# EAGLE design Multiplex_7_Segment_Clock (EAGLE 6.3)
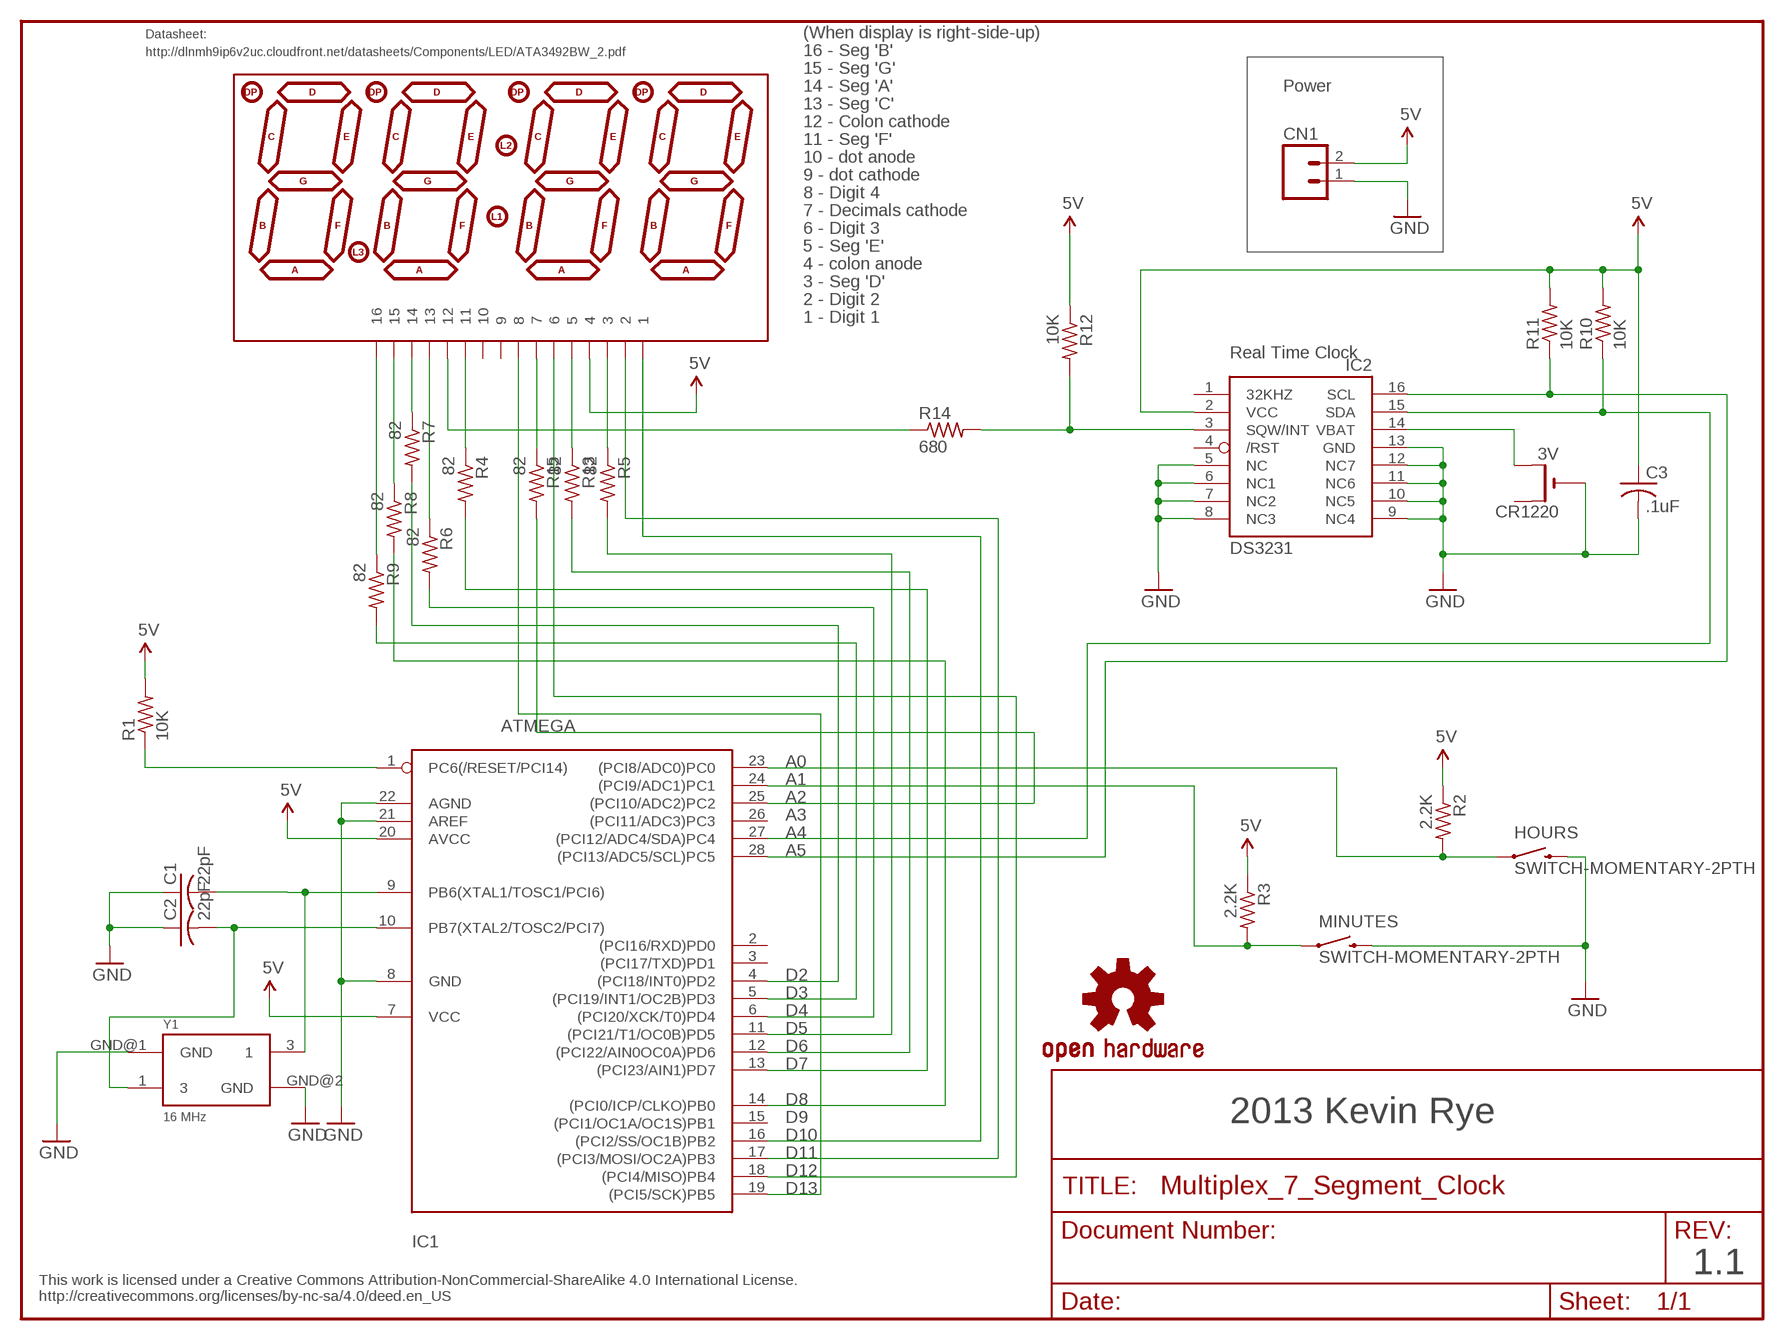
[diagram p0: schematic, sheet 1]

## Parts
C1  22pF  C-USC0805K  [C0805K]
C2  22pF  C-USC0805K  [C0805K]
C3  .1uF  C-USC0805K  [C0805K]
CN1  M02PTH  [1X02]
CR1220  3V  CR1220THM  [CR1220-THM]
HOURS  SWITCH-MOMENTARY-2PTH  [TACTILE-PTH]
IC1  ATMEGA  ATMEGA168PROUND  [DIL28-3-ROUND]
IC2  DS3231  DS3231/SO  [SO16W]
MINUTES  SWITCH-MOMENTARY-2PTH  [TACTILE-PTH]
R1  10K  R-US_R0805  [R0805]
R2  2.2K  R-US_R0805  [R0805]
R3  2.2K  R-US_R0805  [R0805]
R4  82  R-US_R0805  [R0805]
R5  82  R-US_R0805  [R0805]
R6  82  R-US_R0805  [R0805]
R7  82  R-US_R0805  [R0805]
R8  82  R-US_R0805  [R0805]
R9  82  R-US_R0805  [R0805]
R10  10K  R-US_R0805  [R0805]
R11  10K  R-US_R0805  [R0805]
R12  10K  R-US_R0805  [R0805]
R13  82  R-US_R0805  [R0805]
R14  680  R-US_R0805  [R0805]
R15  82  R-US_R0805  [R0805]
U$1  7SEG-4DIGIT  [SPARKFUN_7-SEGMENT-4DIGIT]
U$7  OSHW-LOGOS  [OSHW-LOGO-S]
Y1  16 MHz  OSCILLATOR5X3  [CRYSTAL-SMD-5X3]

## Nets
5V: C3.1 CN1.2 IC1.7(VCC) IC1.20(AVCC) IC2.2(VCC) R1.2 R2.1 R3.1 R10.2 R11.2 R12.1 U$1.4
GND: C1.1 C2.1 C3.2 CN1.1 CR1220.- HOURS.3 IC1.8(GND) IC1.21(AREF) IC1.22(AGND) IC2.5(NC) IC2.6(NC1) IC2.7(NC2) IC2.8(NC3) IC2.9(NC4) IC2.10(NC5) IC2.11(NC6) IC2.12(NC7) IC2.13(GND) MINUTES.3 Y1.GND@1(GND) Y1.GND@2(GND)
N$1: R15.1 U$1.7
N$2: HOURS.1 IC1.23((PCI8/ADC0)PC0) R2.2
N$3: IC1.4((PCI18/INT0)PD2) R7.2
N$4: R9.1 U$1.16
N$5: R8.1 U$1.15
N$6: R14.1 U$1.12
N$7: IC1.5((PCI19/INT1/OC2B)PD3) R9.2
N$8: C2.2 IC1.10(PB7(XTAL2/TOSC2/PCI7)) Y1.1
N$9: IC2.3(SQW/INT) R12.2 R14.2
N$10: C1.2 IC1.9(PB6(XTAL1/TOSC1/PCI6)) Y1.3
N$11: IC1.25((PCI10/ADC2)PC2) R15.2
N$13: CR1220.+2(+1) IC2.14(VBAT)
N$14: IC1.24((PCI9/ADC1)PC1) MINUTES.1 R3.2
N$15: IC1.28((PCI13/ADC5/SCL)PC5) IC2.16(SCL) R11.1
N$17: IC1.6((PCI20/XCK/T0)PD4) R6.2
N$18: IC1.27((PCI12/ADC4/SDA)PC4) IC2.15(SDA) R10.1
N$19: IC1.11((PCI21/T1/OC0B)PD5) R5.2
N$20: IC1.12((PCI22/AIN0OC0A)PD6) R13.2
N$21: IC1.13((PCI23/AIN1)PD7) R4.2
N$22: R6.1 U$1.13
N$23: IC1.14((PCI0/ICP/CLKO)PB0) R8.2
N$24: R7.1 U$1.14
N$25: R4.1 U$1.11
N$27: IC1.16((PCI2/SS/OC1B)PB2) U$1.1
N$28: IC1.17((PCI3/MOSI/OC2A)PB3) U$1.2
N$29: R13.1 U$1.5
N$30: R5.1 U$1.3
N$31: IC1.18((PCI4/MISO)PB4) U$1.6
N$32: IC1.19((PCI5/SCK)PB5) U$1.8
N$35: IC1.1(PC6(/RESET/PCI14)) R1.1
Unconnected: CR1220.+1(+) IC1.2((PCI16/RXD)PD0) IC1.3((PCI17/TXD)PD1) IC1.15((PCI1/OC1A/OC1S)PB1) IC1.26((PCI11/ADC3)PC3) IC2.1(32KHZ) IC2.4(/RST) U$1.9 U$1.10

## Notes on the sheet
- Datasheet: | (When display is right-side-up)
- http://dlnmh9ip6v2uc.cloudfront.net/datasheets/Components/LED/ATA3492BW_2.pdf | 16 - Seg 'B'
- 15 - Seg 'G'
- 14 - Seg 'A' | Power
- 13 - Seg 'C'
- 12 - Colon cathode
- 11 - Seg 'F'
- 10 - dot anode
- 9 - dot cathode
- 8 - Digit 4
- 7 - Decimals cathode
- 6 - Digit 3
- 5 - Seg 'E'
- 4 - colon anode
- 3 - Seg 'D'
- 2 - Digit 2
- 1 - Digit 1
- Real Time Clock
- A0
- A1
- A2
- A3
- A4
- A5
- D2
- D3
- D4
- D5
- D6
- D7
- D8
- D9 | 2013 Kevin Rye
- D10
- D11
- D12
- D13
- 1.1
- This work is licensed under a Creative Commons Attribution-NonCommercial-ShareAlike 4.0 International License.
  http://creativecommons.org/licenses/by-nc-sa/4.0/deed.en_US

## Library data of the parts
C1-C3 = adafruit:C-US: CAPACITOR, American symbol
CN1 = SparkFun w:epaper:M02: Header 2
CR1220 = adafruit:CR1220: CR1216/CR1220/CR1225 12mm 3V lithium coin cell Great for battery packup. Both SMT and THM holders. Note the THM package has the ground pads on both sides of the PCB so that the masks are the same - this reduces the cost
HOURS MINUTES = SparkFun:SWITCH-MOMENTARY-2
IC1 = adafruit:ATMEGA168*P: MICROCONTROLLER 16 kBytes FLASH 1 kBytes SRAM 512 Bytes EEPROM USART 8-channel 10 bit ADC
IC2 = adafruit:DS3231
R1-R15 = adafruit:R-US_: RESISTOR, American symbol
U$1 = sparkfun-4digit-sseg:7SEG-4DIGIT
U$7 = SparkFun:OSHW-LOGO: Open Source Hardware Logo This logo indicates the piece of hardware it is found on incorporates a OSHW license and/or adheres to the definition of open source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
Y1 = SparkFun-FreqCtrl:OSCILLATOR: Generic 5x3 and 7x5 oscillators

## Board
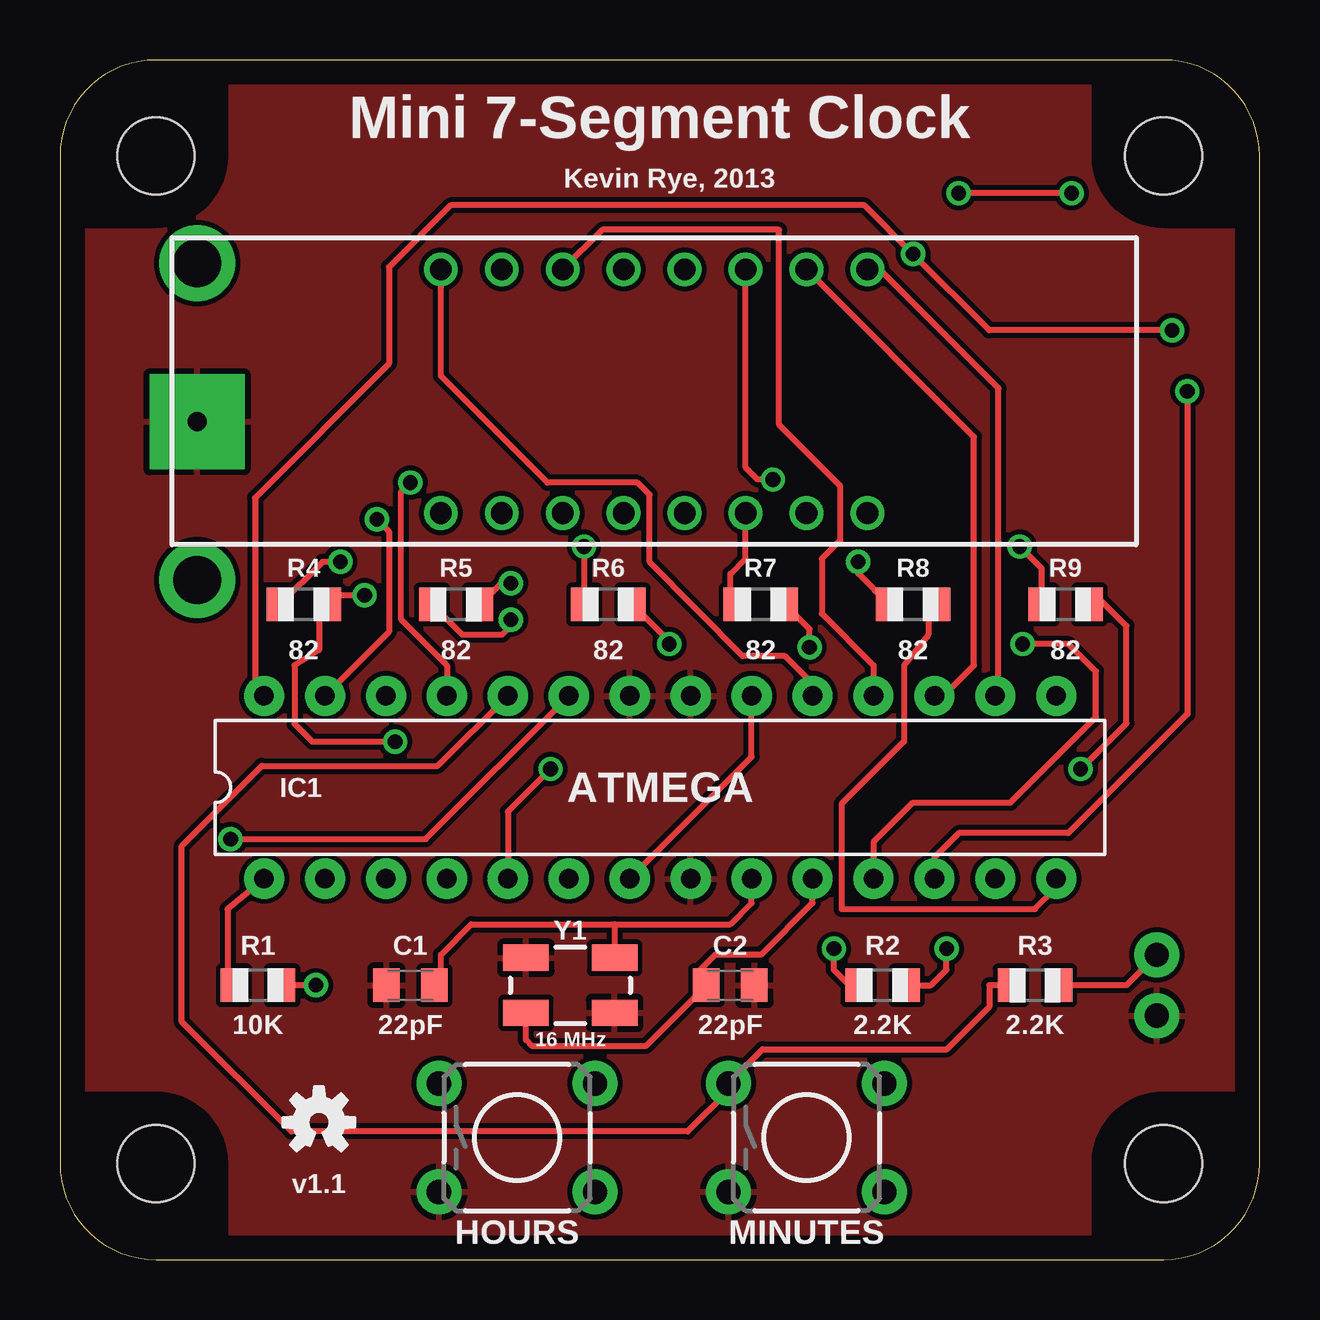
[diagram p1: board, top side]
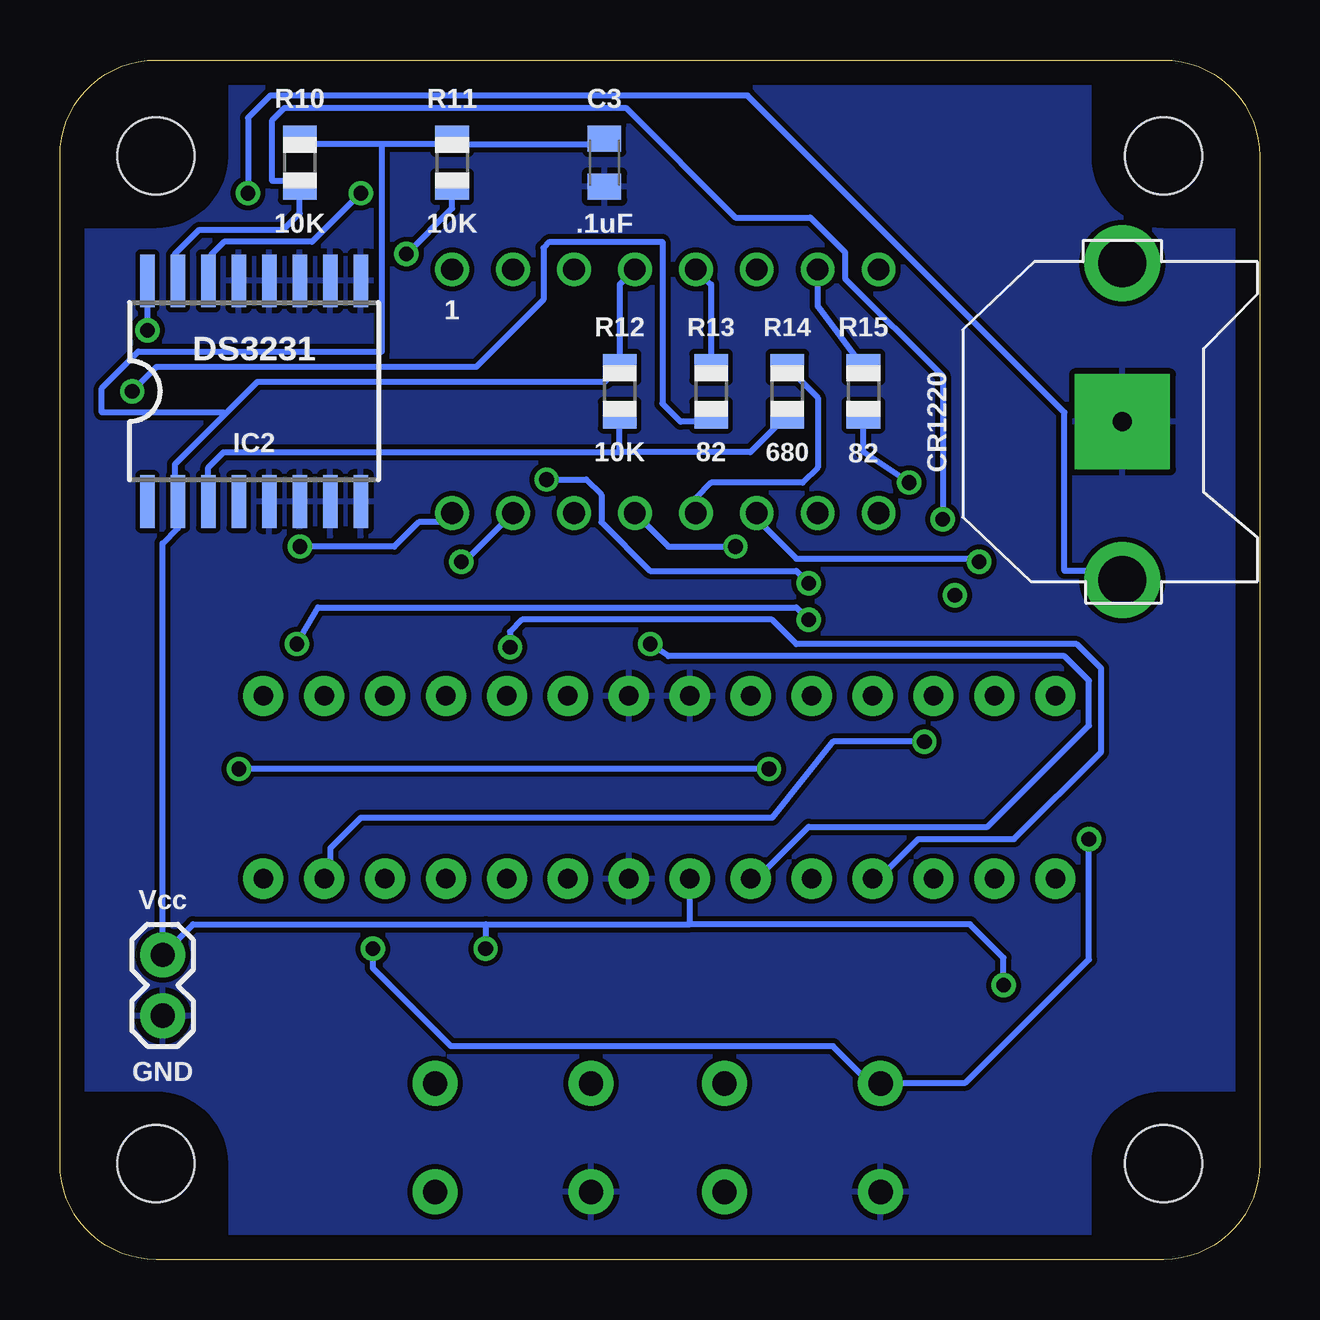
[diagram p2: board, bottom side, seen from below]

Size 50 x 50 mm. Coordinates in mm from the lower left corner, seen from the top.
Copper layers (1*16): Top 0.035mm / dielectric 1.5mm / Bottom 0.035mm
Design rules "default": minimum track width 10mil, minimum drill 24mil, track to track 8mil, track to pad 8mil, pad to pad 8mil, via to via 8mil, smd to smd 8mil, copper to edge 40mil, drill to drill 8mil, minimum pad ring 10mil, minimum via ring 8mil, stop-mask expansion 4mil, vias tented up to drill 0mil, thermal gap 10mil

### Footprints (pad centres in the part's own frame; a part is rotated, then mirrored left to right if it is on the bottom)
C0805K = smd 1.1 x 1.4: 1 -1,0; 2 1,0
1X02 = drill 1.016 pad 1.88: 1 0,0; 2 2.54,0
CR1220-THM = drill 2 pad 3.175: +1 -6.604,0; +2 6.604,0 | drill 0.8 pad 3.962 square: - 0,0
TACTILE-PTH = drill 1.016 pad 1.88: 1 -3.251,2.261; 2 3.251,2.261; 3 -3.251,-2.261; 4 3.251,-2.261
DIL28-3-ROUND = drill 0.813 pad 1.676: 1 -16.51,-3.81; 2 -13.97,-3.81; 3 -11.43,-3.81; 4 -8.89,-3.81; 5 -6.35,-3.81; 6 -3.81,-3.81; 7 -1.27,-3.81; 8 1.27,-3.81; 9 3.81,-3.81; 10 6.35,-3.81; 11 8.89,-3.81; 12 11.43,-3.81; 13 13.97,-3.81; 14 16.51,-3.81; 15 16.51,3.81; 16 13.97,3.81; 17 11.43,3.81; 18 8.89,3.81; 19 6.35,3.81; 20 3.81,3.81; 21 1.27,3.81; 22 -1.27,3.81; 23 -3.81,3.81; 24 -6.35,3.81; 25 -8.89,3.81; 26 -11.43,3.81; 27 -13.97,3.81; 28 -16.51,3.81
SO16W = smd 0.6 x 2.2: 1 -4.445,-4.6; 2 -3.175,-4.6; 3 -1.905,-4.6; 4 -0.635,-4.6; 5 0.635,-4.6; 6 1.905,-4.6; 7 3.175,-4.6; 8 4.445,-4.6; 9 4.445,4.6; 10 3.175,4.6; 11 1.905,4.6; 12 0.635,4.6; 13 -0.635,4.6; 14 -1.905,4.6; 15 -3.175,4.6; 16 -4.445,4.6
R0805 = smd 1.1 x 1.4: 1 -1,0; 2 1,0
SPARKFUN_7-SEGMENT-4DIGIT = drill 0.9: 1 -8.89,-5.08; 2 -6.35,-5.08; 3 -3.81,-5.08; 4 -1.27,-5.08; 5 1.27,-5.08; 6 3.81,-5.08; 7 6.35,-5.08; 8 8.89,-5.08; 9 8.89,5.08; 10 6.35,5.08; 11 3.81,5.08; 12 1.27,5.08; 13 -1.27,5.08; 14 -3.81,5.08; 15 -6.35,5.08; 16 -8.89,5.08
DP5050_V1 = hole 3.2: 4,4; 46,4; 46,46; 4,46
CRYSTAL-SMD-5X3 = smd 1.9 x 1.1: 1 -1.85,-1.15; 3 1.85,1.15; GND@1 -1.85,1.15; GND@2 1.85,-1.15

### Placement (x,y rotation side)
C1  14.61,11.43 0 top
C2  27.94,11.43 180 top
C3  27.3,45.72 270 bottom
CN1  45.72,10.16 90 bottom
CR1220  5.71,34.92 270 bottom
HOURS  19.05,5.08 0 top
IC1  25.02,19.68 0 top
IC2  41.91,36.2 0 bottom
MINUTES  31.11,5.08 0 top
R1  8.26,11.43 0 top
R2  34.29,11.43 0 top
R3  40.64,11.43 180 top
R4  10.16,27.3 0 top
R5  16.51,27.3 180 top
R6  22.86,27.3 0 top
R7  29.21,27.3 0 top
R8  35.56,27.3 0 top
R9  41.91,27.3 0 top
R10  40.01,45.72 90 bottom
R11  33.66,45.72 90 bottom
R12  26.67,36.2 270 bottom
R13  22.86,36.2 270 bottom
R14  19.68,36.2 270 bottom
R15  16.51,36.2 270 bottom
U$1  24.77,36.2 180 top
U$3  [DP5050_V1]  0,0 0 top
U$7  10.79,5.71 0 top
Y1  21.27,11.43 0 top

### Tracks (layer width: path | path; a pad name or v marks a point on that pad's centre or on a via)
5V  (via drill 0.61)
  Top 0.254: v10.67,11.43 R1.2 | 33.53,11.43 R2.1 32.91,11.43 32.26,12.08 v32.26,12.95 | CN1.2 44.45,11.43 R3.1 | IC1.7 28.83,20.95 IC1.20
  Bottom 0.254: C3.1 27.43,46.48 33.53,46.48 R11.2 34.04,46.48 36.58,46.48 | 36.58,46.48 39.62,46.48 R10.2 | 32.26,13.97 44.45,13.97 CN1.2 45.72,29.84 45.09,30.48 IC2.2 | 32.26,13.97 v32.26,12.95 | 45.21,31.24 IC2.2 | 43.12,35.24 41.78,36.58 27.29,36.58 R12.1 26.67,40.64 U$1.4 | 43.12,35.24 45.21,33.14 45.21,31.75 IC2.2 | v10.67,11.43 10.67,12.57 12.06,13.97 23.75,13.97 | 32.26,13.97 23.75,13.97 | 23.75,13.97 IC1.7 | 36.58,46.48 36.58,37.85 46.74,37.85 48.26,36.32 48.26,35.31 43.18,35.31 43.12,35.24
GND
  Top 0.254: Y1.GND@2 23.37,10.41 23.25,10.41
  Bottom 0.254: C3.2 26.92,44.96 26.92,44.85
  pour Bottom: -0.64,50.8 50.8,50.16 50.8,-0.64 -0.64,-0.64
  pour Top: -1.27,51.44 51.44,51.44 51.44,-1.27 -1.27,-1.27
N$1
  Bottom 0.254: R15.1 18.41,39.73 U$1.7
N$2  (via drill 0.61)
  Top 0.254: IC1.23 15.24,17.53 v7.11,17.53 | R2.2 36.31,11.43 36.96,12.08 v36.96,12.95
  Bottom 0.254: v36.96,12.95 36.96,12.14 33.7,8.89 17.78,8.89 16.26,7.37 HOURS.1 15.75,7.37 12.26,7.37 7.11,12.51 v7.11,17.53
N$3  (via drill 0.61)
  Top 0.254: 29.97,27.69 R7.2 31.24,26.27 v31.24,25.53
  Bottom 0.254: IC1.4 15.75,16 14.22,17.53 10.24,17.53 6.6,21.16 6.6,24.64 7.62,25.65 19.3,25.65 20.32,26.67 30.73,26.67 31.24,26.16 v31.24,25.53
N$4  (via drill 0.61)
  Top 0.254: v40.01,29.72 40.91,28.81 R9.1
  Bottom 0.254: v40.01,29.72 36.07,29.72 35.05,30.73 34.04,30.73 U$1.16
N$5  (via drill 0.61)
  Top 0.254: R8.1 33.27,28.59 v33.27,29.08
  Bottom 0.254: v33.27,29.08 33.15,29.08 U$1.15
N$6
  Bottom 0.254: R14.1 18.41,35.92 18.41,33.02 19.05,32.38 22.86,32.38 23.5,31.75 U$1.12
N$7  (via drill 0.61)
  Top 0.254: v42.55,20.45 44.45,22.35 44.45,26.42 43.18,27.69 R9.2 | v20.45,20.45 18.67,18.67 IC1.5
  Bottom 0.254: v20.45,20.45 v42.55,20.45
N$8
  Top 0.254: 19.42,10.53 Y1.1 19.42,9.15 19.68,8.89 24.4,8.89 C2.2 26.67,11.7 26.67,12.06 27.3,12.7 29.21,12.7 31.37,14.86 IC1.10
N$9
  Bottom 0.254: IC2.3 43.81,33.02 43.18,33.66 26.67,33.66 | 26.94,34.92 R12.2 26.67,33.66 | R14.2 21.23,33.66 26.67,33.66
N$10
  Top 0.254: C1.2 15.88,11.43 15.88,12.7 17.14,13.97 23.12,13.97 | 23.12,13.97 27.94,13.97 28.83,14.86 IC1.9 | 23.12,13.97 Y1.3
N$11  (via drill 0.61)
  Top 0.254: v14.61,32.38 14.22,32 14.22,26.67 16.13,24.77 IC1.25
  Bottom 0.254: v14.61,32.38 16.51,33.66 R15.2
N$13  (via drill 0.61)
  Top 0.254: v42.16,44.45 v37.47,44.45
  Bottom 0.254: v42.16,44.45 42.16,47.59 41.24,48.51 21.34,48.51 8.13,35.31 8.13,28.7 6.1,28.7 CR1220.+2 | IC2.14 43.69,40.89 43.69,41.89 43.16,42.42 39.5,42.42 v37.47,44.45
N$14
  Top 0.254: IC1.24 15.75,20.57 8.41,20.57 5.08,17.24 5.08,9.91 9.65,5.33 26.16,5.33 27.86,7.04 MINUTES.1 29.29,8.76 36.97,8.76 38.73,10.53 38.73,11.43 R3.2
N$15  (via drill 0.61)
  Top 0.254: v46.35,38.73 38.73,38.73 v35.56,41.91 33.53,43.94 16.29,43.94 13.72,41.37 13.72,37.34 8.13,31.75 8.13,23.88 IC1.28
  Bottom 0.254: 34.04,44.45 R11.1 33.66,43.81 v35.56,41.91 | IC2.16 v46.35,38.73
N$17  (via drill 0.61)
  Top 0.254: 23.88,27.69 R6.2 25.4,25.77 v25.4,25.65
  Bottom 0.254: v25.4,25.65 24.64,25.15 8.13,25.15 7.11,24.13 7.11,22.26 11.33,18.03 18.8,18.03 20.83,16 IC1.6
N$18  (via drill 0.61)
  Top 0.254: IC1.27 13.72,26.16 13.72,30.35 v13.21,30.86
  Bottom 0.254: 40.13,44.45 R10.1 | IC2.15 45.21,40.89 45.21,41.91 44.2,42.93 40.69,42.93 40.01,43.61 R10.1 | v13.21,30.86 13.21,36.83 17.27,40.89 17.27,41.99 18.72,43.43 21.84,43.43 26.42,48.01 40.64,48.01 41.15,47.5 41.15,44.96 40.13,44.96 R10.1
N$19  (via drill 0.61)
  Top 0.254: v40.13,25.65 42.04,25.65 43.18,24.51 43.18,22.61 39.62,19.05 35.56,19.05 33.91,17.4 IC1.11 | v18.8,26.67 18.8,26.42 18.41,26.04 16.78,26.04 R5.2
  Bottom 0.254: v18.8,26.67 19.3,27.18 39.24,27.18 v40.13,25.65
N$20  (via drill 0.61)
  Top 0.254: v46.99,36.2 46.99,22.74 42.03,17.78 37.47,17.78 36.45,16.76 IC1.12
  Bottom 0.254: v46.99,36.2 45.97,37.21 32.64,37.21 29.84,40.01 29.84,42.16 29.59,42.42 24.89,42.42 24.89,35.69 24.13,34.92 23.13,34.92 R13.2
N$21  (via drill 0.61)
  Top 0.254: R4.2 11.18,27.69 v12.7,27.69 10.79,27.69 10.79,25.4 9.78,24.77 9.78,22.33 10.52,21.59 v13.97,21.59
  Bottom 0.254: v13.97,21.59 17.78,21.59 20.32,18.41 37.47,18.41 38.73,17.14 38.73,16.13 IC1.13
N$22  (via drill 0.61)
  Top 0.254: v21.84,29.72 21.84,28.59 R6.1
  Bottom 0.254: v21.84,29.72 24.64,29.72 U$1.13
N$23
  Top 0.254: 36.58,27.69 R8.2 36.2,26.94 36.2,26.04 35.18,24.77 35.18,21.59 32.58,18.99 32.58,14.61 40.64,14.61 41.53,15.49 IC1.14
N$24
  Top 0.254: R7.1 27.94,27.57 27.94,28.57 28.57,29.21 U$1.14
N$25  (via drill 0.61)
  Top 0.254: v11.68,29.08 10.94,29.08 R4.1
  Bottom 0.254: v11.68,29.08 12.19,29.21 19.3,29.21 20.83,30.73 U$1.11
N$27
  Top 0.254: IC1.16 39.12,23.62 39.12,36.32 34.16,41.27 U$1.1
N$28
  Top 0.254: U$1.2 38.1,34.29 38.1,24.77 36.83,23.5 IC1.17
N$29
  Bottom 0.254: 22.35,37.34 R13.1 22.86,40.64 U$1.5
N$30  (via drill 0.61)
  Top 0.254: v18.8,28.19 18.4,28.19 R5.1 | v29.72,32.51 29.08,32.51 28.57,33.02 U$1.3
  Bottom 0.254: v18.8,28.19 19.3,28.7 25.4,28.7 27.43,30.73 27.43,31.88 28.07,32.51 v29.72,32.51
N$31
  Top 0.254: IC1.18 33.91,24.77 31.75,26.92 31.75,29.21 32.51,29.97 32.51,32.26 29.97,34.8 29.97,42.93 22.61,42.93 U$1.6
N$32
  Top 0.254: IC1.19 31.37,24 30.23,25.15 28.45,25.15 24.57,29.08 24.57,31.88 24.07,32.38 20.32,32.38 15.88,36.83 U$1.8
N$35
  Top 0.254: 7.62,11.43 R1.1 6.99,11.7 6.99,14.61 IC1.1

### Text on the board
Unrouted: This work is licensed under a Creative Commons Attribution-NonCommercial-ShareAlike 4.0 International License. / http://creativecommons.org/licenses/by-nc-sa/4.0/deed.en_US
bPlace: 1
tNames: Mini 7-Segment Clock | Kevin Rye, 2013 | v1.1
bNames: Vcc | GND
